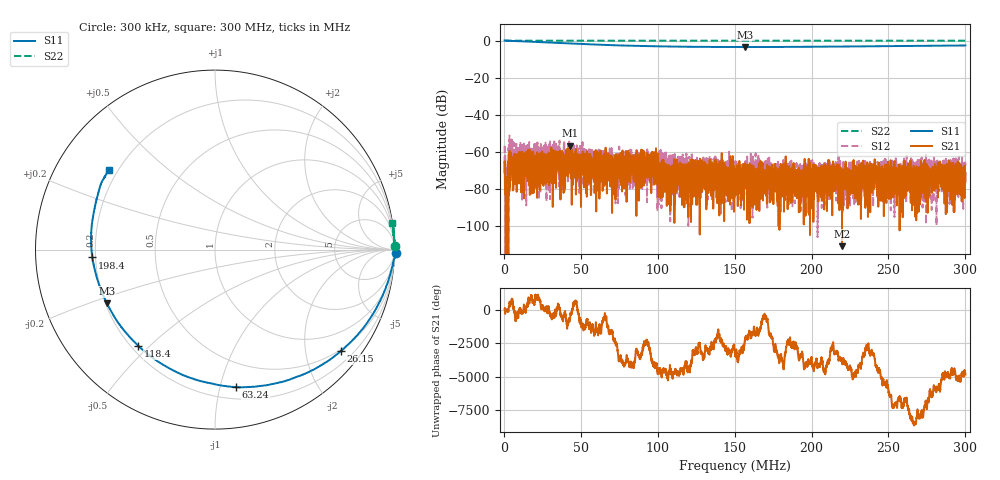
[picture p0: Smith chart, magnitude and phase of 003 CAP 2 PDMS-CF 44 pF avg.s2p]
!  26/06/2025  14:55:21
! Ref Plane: 0.000 mm
# MHZ S MA R  50
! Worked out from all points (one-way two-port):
!   4001 points, 300 kHz to 300 MHz, reference 50 ohm
!   highest |S21| = -56.75 dB at 42.71 MHz (marker M1); lowest = -111.0 dB at 219.8 MHz (marker M2)
!   lowest |S11| = -3.5 dB at 156.8 MHz (marker M3), VSWR 5.10, Z = 10.3 - j11.2 ohm
!   |S11| at or under -10 dB: nowhere
!   |S22| runs from 0.0 to 0.1 dB; largest |S21 - S12| = 0.0033
!   S11 on the Smith chart (normalised r, x): 300 kHz: -39, -74; 26.15 MHz: 0.46, -2.78; 63.24 MHz: 0.29, -1.12; 118.4 MHz: 0.23, -0.46; 198.4 MHz: 0.19, -0.03; 300 MHz: 0.16, +0.32
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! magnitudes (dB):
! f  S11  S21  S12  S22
! 300 kHz  0.1  -71.1  -66.3  0.0
! 2.398 MHz  -0.1  -85.8  -  0.0
! 4.346 MHz  -0.1  -66.5  -57.8  0.0
! 26.15 MHz  -0.9  -74.9  -63.0  0.0
! 42.71 MHz  -1.5  -56.8  -61.7  0.0
! 50.28 MHz  -1.8  -66.5  -64.4  0.0
! 63.24 MHz  -2.2  -65.8  -63.0  0.0
! 73.06 MHz  -2.5  -63.2  -82.3  0.0
! 76.13 MHz  -2.6  -63.3  -63.3  0.0
! 97.41 MHz  -3.0  -65.5  -71.1  0.0
! 100.3 MHz  -3.1  -82.5  -76.6  0.0
! 118.4 MHz  -3.3  -74.3  -76.0  0.0
! 150.2 MHz  -3.4  -71.5  -69.7  0.0
! 156.8 MHz  -3.5  -66.5  -68.6  0.0
! 198.4 MHz  -3.3  -69.7  -72.1  0.0
! 200.1 MHz  -3.3  -71.6  -69.4  0.0
! 219.8 MHz  -3.2  -111.0  -69.9  0.0
! 250.1 MHz  -3.0  -78.5  -73.4  0.0
! 289.2 MHz  -2.7  -68.3  -81.2  0.0
! 293.7 MHz  -2.6  -66.4  -63.6  0.0
! 297.8 MHz  -2.6  -74.5  -62.9  0.0
! 300 MHz  -2.6  -76.2  -66.2  0.0
